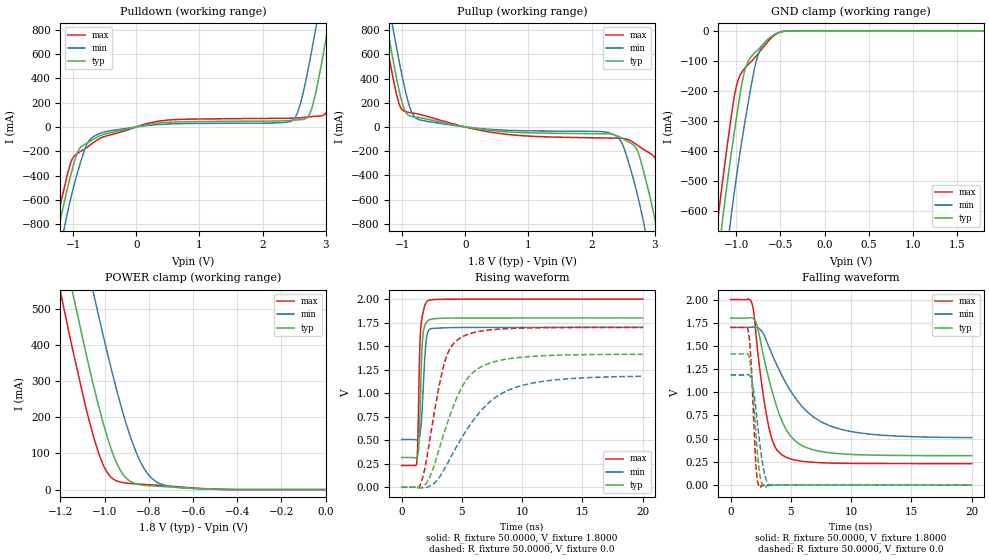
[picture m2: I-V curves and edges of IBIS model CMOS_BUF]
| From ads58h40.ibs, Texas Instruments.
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|   Model cmos_data_high1
|   Model CMOS_BUF
[Model]  CMOS_BUF
Model_type 3-state
Polarity   Non-Inverting
Enable   Active-High
Vmeas =  1.2V
C_comp   2.5000pF   2.2500pF   2.7500pF
[Temperature Range]   25.0000   0.1250k   -40.0000
[Voltage Range]   1.8000V   1.7000V   2.0000V
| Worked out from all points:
|   slope of the pulldown table from 0 to 0.27 V, typ, clamps not added: 10.1 ohm
|   slope of the pullup table from 0 to 0.27 V, typ, clamps not added: 12.7 ohm
|   GND clamp passes 1 mA (typ) near -0.45 V on its own axis
|   POWER clamp passes 1 mA (typ) near -0.50 V on its own axis
|   rising waveform, R_fixture 50.0000, V_fixture 1.8000: 20-80 % time 224ps typ, 303ps min, 202ps max; typ from 0.316 V to 1.8 V
|   rising waveform, R_fixture 50.0000, V_fixture 0.0: 20-80 % time 2.5ns typ, 3.94ns min, 1.52ns max; typ from 0 V to 1.41 V
|   falling waveform, R_fixture 50.0000, V_fixture 1.8000: 20-80 % time 2ns typ, 3.46ns min, 1.14ns max; typ from 1.8 V to 0.317 V
|   falling waveform, R_fixture 50.0000, V_fixture 0.0: 20-80 % time 485ps typ, 664ps min, 363ps max; typ from 1.42 V to 0 V
[Pulldown]
|Voltage   I(typ)   I(min)   I(max)
-1.8V     -2.54A     -2.76A     -2.411A
-1.29V    -999.1mA   -1.236A    -863.8mA
-1.19V    -735mA     -959.6mA   -612mA
-910mV    -186.8mA   -340.3mA   -209.6mA
-570mV    -71.06mA   -51.78mA   -92.64mA
2.48V     55.09mA    55.76mA    71.97mA
2.75V     110.1mA    548.1mA    83.31mA
2.86V     324.6mA    858.6mA    88.04mA
2.98V     652.7mA    1.215A     101.6mA
3.05V     859.5mA    1.428A     175.7mA
3.32V     1.694A     2.262A     915.1mA
3.6V      2.576A     3.128A     1.796A
[Pullup]
|Voltage   I(typ)   I(min)   I(max)
-1.8V     2.578A     2.82A      2.436A
-1.42V    1.383A     1.646A     1.228A
-1.21V    744mA      1.008A     589.4mA
-1.14V    543.2mA    803.4mA    394.8mA
-1.03V    262.6mA    498.9mA    167.6mA
-890mV    93.4mA     182.4mA    120.1mA
-320mV    32.01mA    22.75mA    44.27mA
2.4V      -72.71mA   -79.61mA   -92.65mA
2.82V     -358.3mA   -777.1mA   -184.5mA
3.03V     -834.6mA   -1.35A     -283.6mA
3.29V     -1.584A    -2.126A    -864.1mA
3.6V      -2.539A    -3.06A     -1.784A
[GND_clamp]
|Voltage   I(typ)   I(min)   I(max)
-1.8V     -2.535A    -2.755A    -2.405A
-1.26V    -904.2mA   -1.144A    -765mA
-1.2V     -743.7mA   -977.4mA   -610.1mA
-1.15V    -618.5mA   -844.4mA   -490.6mA
-1.1V     -502.5mA   -718.1mA   -379mA
-1.05V    -395.4mA   -600mA     -272.5mA
-1V       -295.2mA   -491.3mA   -186.5mA
-890mV    -118.8mA   -283.2mA   -120.3mA
-790mV    -73.21mA   -120.7mA   -89.43mA
-740mV    -58.88mA   -70.25mA   -71.95mA
-590mV    -17.15mA   -16.54mA   -20.34mA
1.8V      478pA      53.04nA    24.72pA
[POWER_clamp]
|Voltage   I(typ)   I(min)   I(max)
-1.8V     2.573A     2.816A     2.431A
-1.22V    764.6mA    1.032A     605.2mA
-1.15V    559.4mA    825.3mA    401.5mA
-1.05V    287.1mA    542.1mA    145.6mA
-1V       169.9mA    409.1mA    59.68mA
-950mV    79.48mA    285.7mA    25.24mA
-910mV    36.72mA    197.4mA    18.72mA
-850mV    14.76mA    92.42mA    15.41mA
-810mV    11.28mA    47.56mA    13.94mA
-760mV    9.358mA    19.44mA    12.15mA
-580mV    2.857mA    2.498mA    3.804mA
0V        478pA      21.25nA    33.72pA
[Ramp]
| variable   typ   min   max
dV/dt_r  0.8482/2.4950n   0.7082/3.9383n   1.0194/1.5181n
dV/dt_f  0.8900/1.9994n   0.7134/3.4549n   1.0613/1.1436n
R_load = 50.0000
[Rising Waveform]
R_fixture= 50.0000
V_fixture= 1.8000
V_fixture_min= 1.7000
V_fixture_max= 2.0000
|time   V(typ)   V(min)   V(max)
0s        316.5mV    508.1mV    231.2mV
1.26ns    316.5mV    501.3mV    257.1mV
1.34ns    334.6mV    497.7mV    438.4mV
1.42ns    414.9mV    510mV      905.6mV
1.5ns     658mV      529.1mV    1.41V
1.58ns    1.012V     601.9mV    1.665V
1.78ns    1.623V     1.011V     1.851V
2ns       1.738V     1.499V     1.954V
2.18ns    1.769V     1.651V     1.982V
20ns      1.8V       1.7V       2V
[Rising Waveform]
R_fixture= 50.0000
V_fixture= 0.0
V_fixture_min= 0.0
V_fixture_max= 0.0
|time   V(typ)   V(min)   V(max)
0s        1nV        49.03nV    169.1pV
1.56ns    -6.284mV   -1.39mV    30.72mV
1.92ns    23.46mV    -5.958mV   191.9mV
2.38ns    118.4mV    15.38mV    532.2mV
3.48ns    556.1mV    176.4mV    1.285V
4.04ns    771.5mV    308.5mV    1.478V
4.82ns    1.016V     489mV      1.583V
6.38ns    1.263V     781.8mV    1.655V
9.3ns     1.373V     1.055V     1.689V
20ns      1.414V     1.18V      1.699V
[Falling Waveform]
R_fixture= 50.0000
V_fixture= 1.8000
V_fixture_min= 1.7000
V_fixture_max= 2.0000
|time   V(typ)   V(min)   V(max)
0s        1.8V       1.7V       2V
1.76ns    1.802V     1.704V     1.963V
1.96ns    1.786V     1.704V     1.827V
2.2ns     1.719V     1.699V     1.505V
3.12ns    1.175V     1.511V     659.3mV
3.58ns    950.1mV    1.368V     444.4mV
4.28ns    686.4mV    1.176V     323.2mV
5.8ns     435.8mV    867.3mV    258.9mV
8.64ns    342.1mV    620.7mV    235.9mV
20ns      316.6mV    511.1mV    231.2mV
[Falling Waveform]
R_fixture= 50.0000
V_fixture= 0.0
V_fixture_min= 0.0
V_fixture_max= 0.0
|time   V(typ)   V(min)   V(max)
0s        1.415V     1.187V     1.699V
1.34ns    1.418V     1.19V      1.701V
1.48ns    1.402V     1.189V     1.651V
1.7ns     1.248V     1.151V     1.329V
2.12ns    526.2mV    798mV      185.7mV
2.24ns    331.8mV    655.1mV    35.42mV
2.42ns    122.8mV    451.7mV    -25.76mV
2.84ns    -30.48mV   111.3mV    1.222mV
3.26ns    -5.698mV   -4.298mV   518.8uV
20ns      74.63nV    892.5nV    6.313nV
